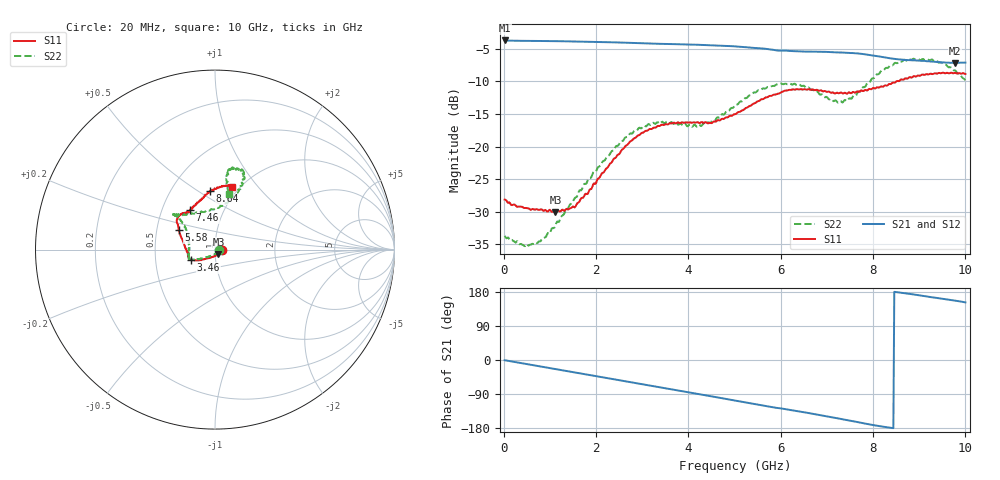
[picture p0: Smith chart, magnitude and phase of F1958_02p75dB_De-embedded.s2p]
! Integrated Device Technology
! Corporate Headquarters
! 6024 Silver Creek Valley Road
! San Jose, CA 95138  USA
! Phone:  1-408-284-8200
! Toll Free:  1-800-223-1366
! Webpage:  http://www.idt.com/
! Timing and RF Division
! 515 Groton Road, Suite 102
! Westford, MA 01886-6024
! Device:  F1958
! Description: 7-bit 0.25 dB Digital Step Attenuator
! Frequency:  0.001 -  6.000 GHz
! Package:  4x4 mm Thin QFN Plastic Package: 24 pin
! Ports:  2 RF, 12 DC
!  Pin  1  = D0
!  Pin  2  = VDD
!  Pin  3  = VMODE
!  Pin  4  = GND
!  Pin  5  = RF1  =  Port 1
!  Pin  6  = GND
!  Pin  7  = GND
!  Pin  8  = GND
!  Pin  9  = GND
!  Pin 10  = GND
!  Pin 11  = GND
!  Pin 12  = GND
!  Pin 13  = GND
!  Pin 14  = RF2  =  Port 2
!  Pin 15  = GND
!  Pin 16  = LE
!  Pin 17  = CLK
!  Pin 18  = DATA
!  Pin 19  = D6
!  Pin 20  = D5
!  Pin 21  = D4
!  Pin 22  = D3
!  Pin 23  = D2
!  Pin 24  = D1
! State:  11
! Atten State:  2.75 dB
! Voltage:  +3.30 Volts
! Current:  0.258 mA
! Data:  The device was measured on a F1958 evaluation board which has
!  individual transmission lines to the RF pins.  Data was collected
!  using a calibrated network analyzer.  The evaluation board was
!  de-embedded using Automatic Fixture Removal (AFR).
!  The reference plane is the edge of the package pin.
! Misc:
!  Action Tracker AT0419
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# GHz S dB R 50
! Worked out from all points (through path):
!   500 points, 20 MHz to 10 GHz, reference 50 ohm
!   highest |S21| = -3.72 dB at 20 MHz (marker M1); lowest = -7.2 dB at 9.78 GHz (marker M2)
!   group delay of S21, straight-line fit = 58.5 ps
!   lowest |S11| = -30.0 dB at 1.12 GHz (marker M3), VSWR 1.07, Z = 51.9 - j2.61 ohm
!   |S11| at or under -10 dB: start of sweep to 8.506 GHz
!   |S22| runs from -35.3 to -6.5 dB; largest |S21 - S12| = 0.0019
!   S11 on the Smith chart (normalised r, x): 20 MHz: 1.08, -0.00; 3.46 GHz: 0.76, -0.09; 5.58 GHz: 0.65, +0.15; 7.46 GHz: 0.70, +0.33; 8.64 GHz: 0.77, +0.56; 10 GHz: 0.92, +0.74
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0.02  -28.12 -3.3  -3.72 -0.6  -3.72 -0.5  -33.69 -6.2
0.56  -29.55 -17.4  -3.79 -12.0  -3.79 -12.0  -35.07 -37.0
0.76  -29.70 -26.7  -3.80 -16.2  -3.80 -16.2  -34.54 -53.1
1.12  -30.02 -52.8  -3.83 -23.9  -3.83 -23.9  -32.15 -90.9
1.52  -29.23 -87.9  -3.88 -32.4  -3.88 -32.4  -28.12 -120.1
1.7  -27.85 -100.9  -3.90 -36.2  -3.90 -36.2  -26.46 -128.9
2.6  -20.28 -143.3  -4.06 -55.4  -4.05 -55.4  -18.95 -151.6
2.96  -18.10 -151.4  -4.14 -63.1  -4.13 -63.2  -17.16 -154.8
3.36  -16.84 -156.1  -4.24 -71.6  -4.24 -71.7  -16.38 -159.8
3.46  -16.69 -157.2  -4.25 -73.7  -4.26 -73.8  -16.31 -161.3
4.32  -16.34 -169.4  -4.41 -92.0  -4.42 -92.0  -16.48 168.3
5.02  -15.01 168.6  -4.63 -107.3  -4.65 -107.2  -13.60 143.6
5.58  -12.75 151.8  -4.96 -119.3  -4.97 -119.3  -11.26 138.3
6.04  -11.58 143.8  -5.28 -128.4  -5.29 -128.3  -10.41 139.5
6.68  -11.24 133.6  -5.44 -141.5  -5.46 -141.4  -11.26 133.9
7.2  -11.78 126.7  -5.55 -153.1  -5.56 -153.0  -12.94 109.5
7.46  -11.75 122.2  -5.62 -159.1  -5.62 -159.0  -12.80 89.5
8.34  -10.43 102.1  -6.42 -178.2  -6.42 -178.3  -7.81 67.0
8.64  -9.74 94.7  -6.67 176.9  -6.68 177.0  -6.88 69.1
9.28  -8.88 80.3  -6.96 165.4  -6.97 165.4  -6.64 79.0
9.78  -8.69 75.4  -7.17 156.6  -7.19 156.6  -8.33 79.7
10  -8.85 74.9  -7.12 151.9  -7.15 152.1  -9.83 75.6
